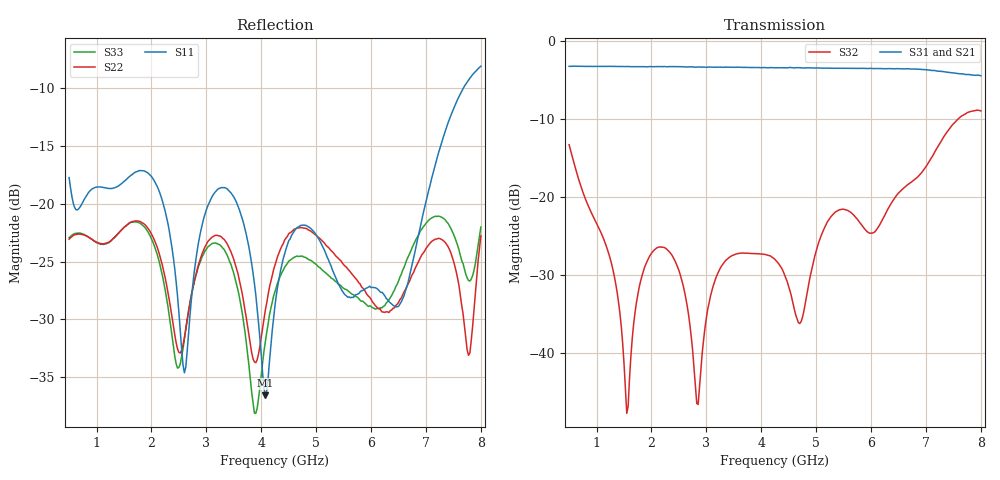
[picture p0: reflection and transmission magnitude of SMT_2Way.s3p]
! Created Tue Jan 09 16:02:54 2018
# hz S ma R 50
! 3 Port Network Data from SP1.SP block
! freq  magS11  angS11  magS12  angS12  magS13  angS13
!  magS21  angS21
!  magS22  angS22  magS23  angS23
!  magS31  angS31  magS32  angS32
!  magS33  angS33
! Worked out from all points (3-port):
!   301 points, 500 MHz to 8 GHz, reference 50 ohm
!   strongest paths, dB at 500 MHz, 2.375 GHz, 4.25 GHz, 6.125 GHz, 8 GHz:
!     S31: -3.3, -3.3, -3.5, -3.6, -4.5
!     S21: -3.3, -3.3, -3.5, -3.6, -4.5
!     S32: -13.3, -27.5, -28.0, -24.0, -9.0
!   lowest |S11| = -36.6 dB at 4.075 GHz (marker M1), VSWR 1.03, Z = 51.2 + j0.884 ohm
!   |S11| at or under -10 dB: start of sweep to 7.681 GHz
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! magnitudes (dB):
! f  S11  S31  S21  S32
! 500 MHz  -17.7  -3.3  -3.3  -13.3
! 1.55 GHz  -17.9  -3.3  -3.3  -47.8
! 2.025 GHz  -17.8  -3.3  -3.3  -27.0
! 2.6 GHz  -34.6  -3.4  -3.4  -32.1
! 2.825 GHz  -24.3  -3.4  -3.4  -46.5
! 3.525 GHz  -19.6  -3.4  -3.4  -27.4
! 4.075 GHz  -36.6  -3.5  -3.5  -27.4
! 4.25 GHz  -28.8  -3.5  -3.5  -28.0
! 6.5 GHz  -28.9  -3.6  -3.6  -19.5
! 8 GHz  -8.1  -4.5  -4.5  -9.0
